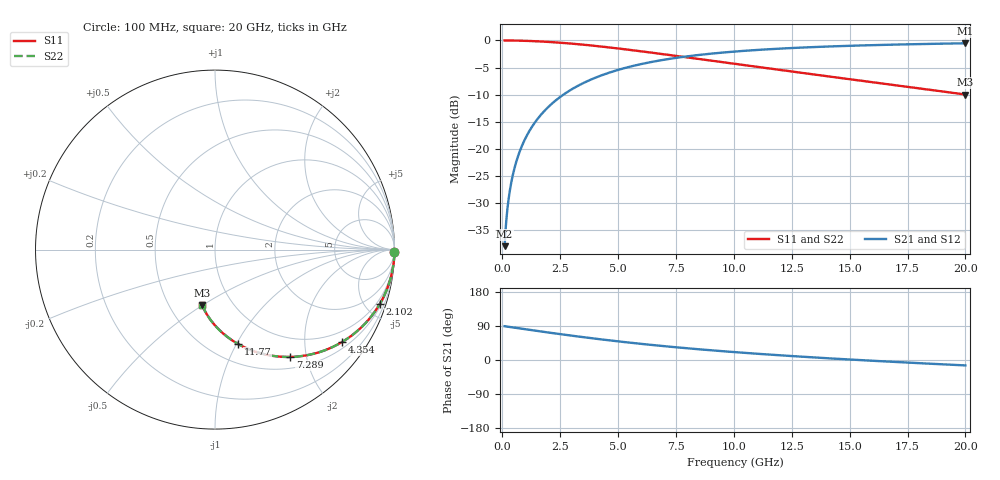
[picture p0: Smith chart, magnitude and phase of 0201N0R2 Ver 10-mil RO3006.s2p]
# GHz S MA R 50
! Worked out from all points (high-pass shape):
!   1601 points, 100 MHz to 20 GHz, reference 50 ohm
!   highest |S21| = -0.52 dB at 20 GHz (marker M1); lowest = -38.0 dB at 100 MHz (marker M2)
!   |S21| within 3 dB of the highest: 7.038 GHz to end of sweep
!   lowest |S11| = -10.0 dB at 20 GHz (marker M3), VSWR 1.93, Z = 36.2 - j24.8 ohm
!   |S11| at or under -10 dB: nowhere
!   |S22| runs from -10.0 to 0.0 dB; largest |S21 - S12| = 0
!   S11 on the Smith chart (normalised r, x): 100 MHz: open; 2.102 GHz: 0.67, -6.12; 4.354 GHz: 0.67, -2.93; 7.289 GHz: 0.67, -1.72; 11.77 GHz: 0.68, -1.02; 20 GHz: 0.72, -0.50
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0.1  0.9999 -0.9  0.0126 89.1  0.0126 89.1  0.9999 -0.9
0.14975  0.9998 -1.3  0.01887 88.7  0.01887 88.7  0.9998 -1.3
0.2616875  0.9994 -2.3  0.03296 87.7  0.03296 87.7  0.9994 -2.3
0.3611875  0.999 -3.2  0.04547 86.8  0.04547 86.8  0.999 -3.2
0.5104375  0.9979 -4.5  0.06419 85.5  0.06419 85.5  0.9979 -4.5
0.7094375  0.996 -6.3  0.08905 83.7  0.08905 83.7  0.996 -6.3
0.970625  0.9925 -8.6  0.1214 81.4  0.1214 81.4  0.9925 -8.6
1.281562  0.9871 -11.3  0.1595 78.7  0.1595 78.7  0.9871 -11.3
1.654688  0.9788 -14.5  0.2042 75.4  0.2042 75.4  0.9788 -14.5
2.102438  0.9663 -18.4  0.2563 71.6  0.2563 71.6  0.9663 -18.4
2.711875  0.9457 -23.4  0.3237 66.5  0.3237 66.5  0.9457 -23.4
3.420812  0.9173 -29.1  0.3965 60.8  0.3965 60.8  0.9173 -29.1
4.353625  0.875 -36.1  0.4821 53.8  0.4821 53.8  0.875 -36.1
5.497875  0.8189 -44.0  0.5714 45.8  0.5714 45.8  0.8189 -44.0
6.741625  0.757 -51.8  0.6502 38.0  0.6502 38.0  0.757 -51.8
7.288875  0.7304 -55.0  0.6797 34.8  0.6797 34.8  0.7304 -55.0
8.657  0.6668 -62.3  0.7414 27.4  0.7414 27.4  0.6668 -62.3
10.05  0.6073 -68.9  0.7902 20.7  0.7902 20.7  0.6073 -68.9
11.76638  0.5418 -76.2  0.8356 13.3  0.8356 13.3  0.5418 -76.2
13.37081  0.4878 -82.3  0.8676 7.1  0.8676 7.1  0.4878 -82.3
16.69162  0.3938 -93.5  0.9131 -4.3  0.9131 -4.3  0.3938 -93.5
20  0.3168 -103.1  0.9415 -14.3  0.9415 -14.3  0.3168 -103.1
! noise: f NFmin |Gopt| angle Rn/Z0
0.1  0.002  0.9876  0.7988  0.03684
2.301  0.005621  0.8471  6.837  0.00779
4.515  0.008438  0.7957  10.28  0.00847
6.729  0.0109  0.7648  13.69  0.009287
8.943  0.01317  0.7429  17.12  0.01005
11.14  0.01529  0.7262  20.54  0.01075
13.36  0.01733  0.7129  23.98  0.01141
15.57  0.01932  0.7021  27.39  0.01202
17.79  0.02126  0.6933  30.79  0.01259
20  0.02317  0.686  34.15  0.01313
